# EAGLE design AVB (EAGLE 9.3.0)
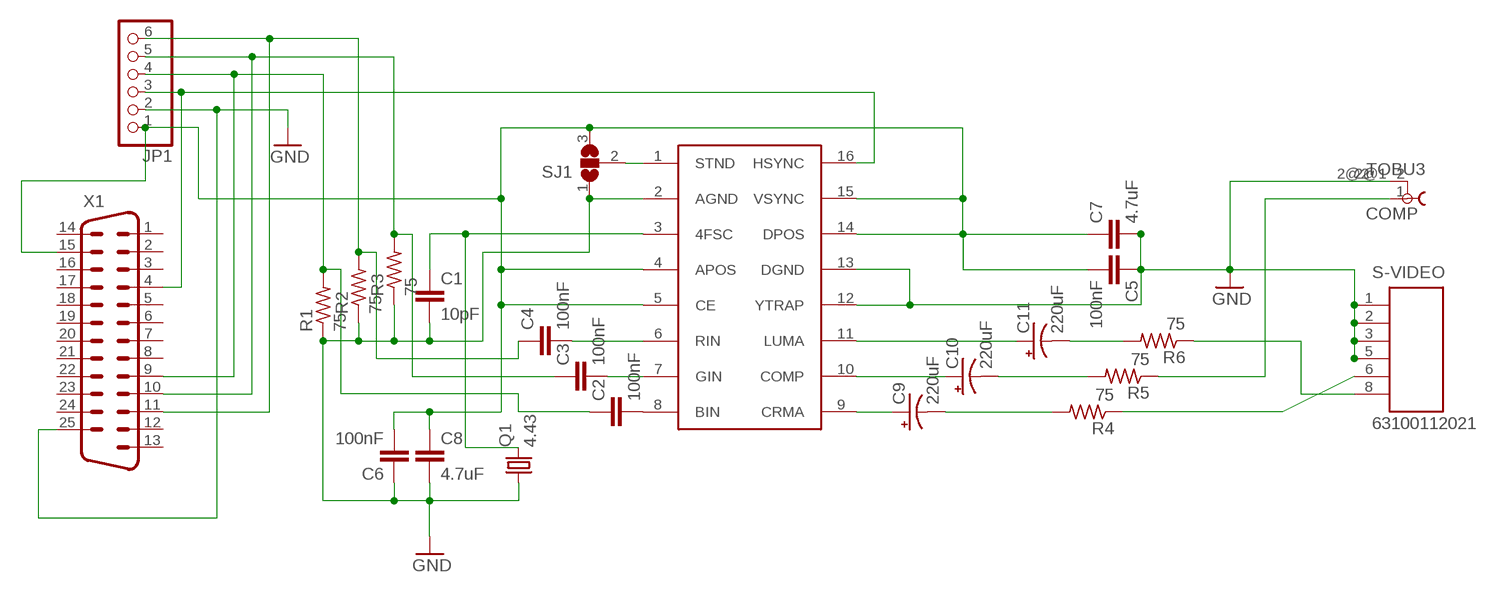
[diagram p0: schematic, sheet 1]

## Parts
C1  10pF  C-EUC0603  [C0603]
C2  100nF  C-EUC0603  [C0603]
C3  100nF  C-EUC0603  [C0603]
C4  100nF  C-EUC0603  [C0603]
C5  100nF  C-EUC0603  [C0603]
C6  100nF  C-EUC0603  [C0603]
C7  4.7uF  C-EUC0603  [C0603]
C8  4.7uF  C-EUC0603  [C0603]
C9  220uF  CPOL-USCT6032  [CT6032]
C10  220uF  CPOL-USCT6032  [CT6032]
C11  220uF  CPOL-USCT6032  [CT6032]
COMP  TOBU3  [TOBU3]
JP1  PINHD-1X6  [1X06]
Q1  4.43  CRYSTALHC49S  [HC49/S]
R1  75  R-US_R0805  [R0805]
R2  75  R-US_R0805  [R0805]
R3  75  R-US_R0805  [R0805]
R4  75  R-US_R0805  [R0805]
R5  75  R-US_R0805  [R0805]
R6  75  R-US_R0805  [R0805]
S-VIDEO  63100112021  [63100112021]
SJ1  SJ2W  [SJ_2]
U1  AD725  [SO16W]
X1  M25D  [M25D]

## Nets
GND: C1.2 C5.1 C6.1 C7.2 C8.2 COMP.2 JP1.2 Q1.1 R1.1 R2.1 R3.1 S-VIDEO.1 S-VIDEO.2 S-VIDEO.3 S-VIDEO.5 SJ1.1 U1.2(AGND) U1.12(YTRAP) U1.13(DGND) X1.25
N$1: C4.1 JP1.6 R2.2 X1.11
N$2: SJ1.2 U1.1(STND)
N$3: C5.2 C6.2 C7.1 C8.1 JP1.1 SJ1.3 U1.4(APOS) U1.5(CE) U1.14(DPOS) U1.15(VSYNC) X1.15
N$4: C4.2 U1.6(RIN)
N$6: JP1.3 U1.16(HSYNC) X1.4
N$7: C3.2 U1.7(GIN)
N$8: C2.2 U1.8(BIN)
N$9: COMP.1 R5.1
N$10: C3.1 JP1.5 R3.2 X1.10
N$11: R6.1 S-VIDEO.8
N$12: R4.1 S-VIDEO.6
N$14: C2.1 JP1.4 R1.2 X1.9
N$18: C1.1 Q1.2 U1.3(4FSC)
N$23: C11.+ U1.11(LUMA)
N$24: C10.+ U1.10(COMP)
N$25: C9.+ U1.9(CRMA)
N$26: C11.- R6.2
N$27: C10.- R5.2
N$28: C9.- R4.2
Unconnected: COMP.2@1 COMP.2@2 X1.1 X1.2 X1.3 X1.5 X1.6 X1.7 X1.8 X1.12 X1.13 X1.14 X1.16 X1.17 X1.18 X1.19 X1.20 X1.21 X1.22 X1.23 X1.24

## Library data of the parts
C1-C8 = resistor:C-EU: CAPACITOR, European symbol
C9-C11 = adafruit:CPOL-US: POLARIZED CAPACITOR, American symbol
COMP = con-hirschmann:TOBU3: Female Cinch CONNECTOR ( RCA Jack )
JP1 = pinhead:PINHD-1X6: PIN HEADER
Q1 = crystal:CRYSTAL: CRYSTAL; OC_FARNELL: 1667008; OC_NEWARK: unknown
R1-R6 = resistor:R-US_: RESISTOR, American symbol
S-VIDEO = Wuerth_Elektronik_eiCan_Communication_Connectors_v2.2:63100112021: WR-COM Horizontal Shielded Mini DIN, 6 Pins
SJ1 = jumper:SJ2W: SMD solder JUMPER
U1 = ad725:AD725
X1 = con-subd:M25: SUB-D; OC_FARNELL: unknown; OC_NEWARK: unknown

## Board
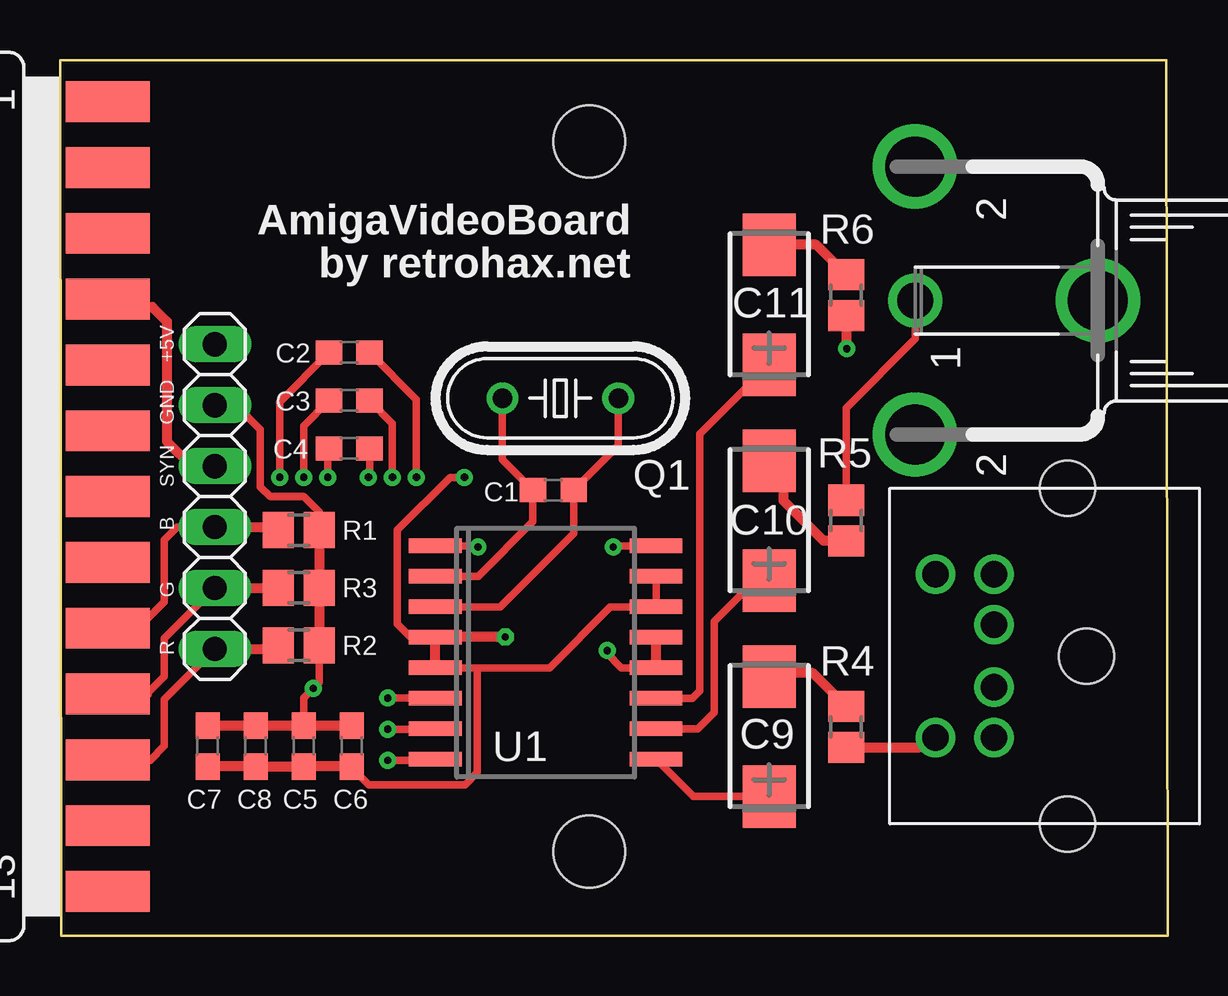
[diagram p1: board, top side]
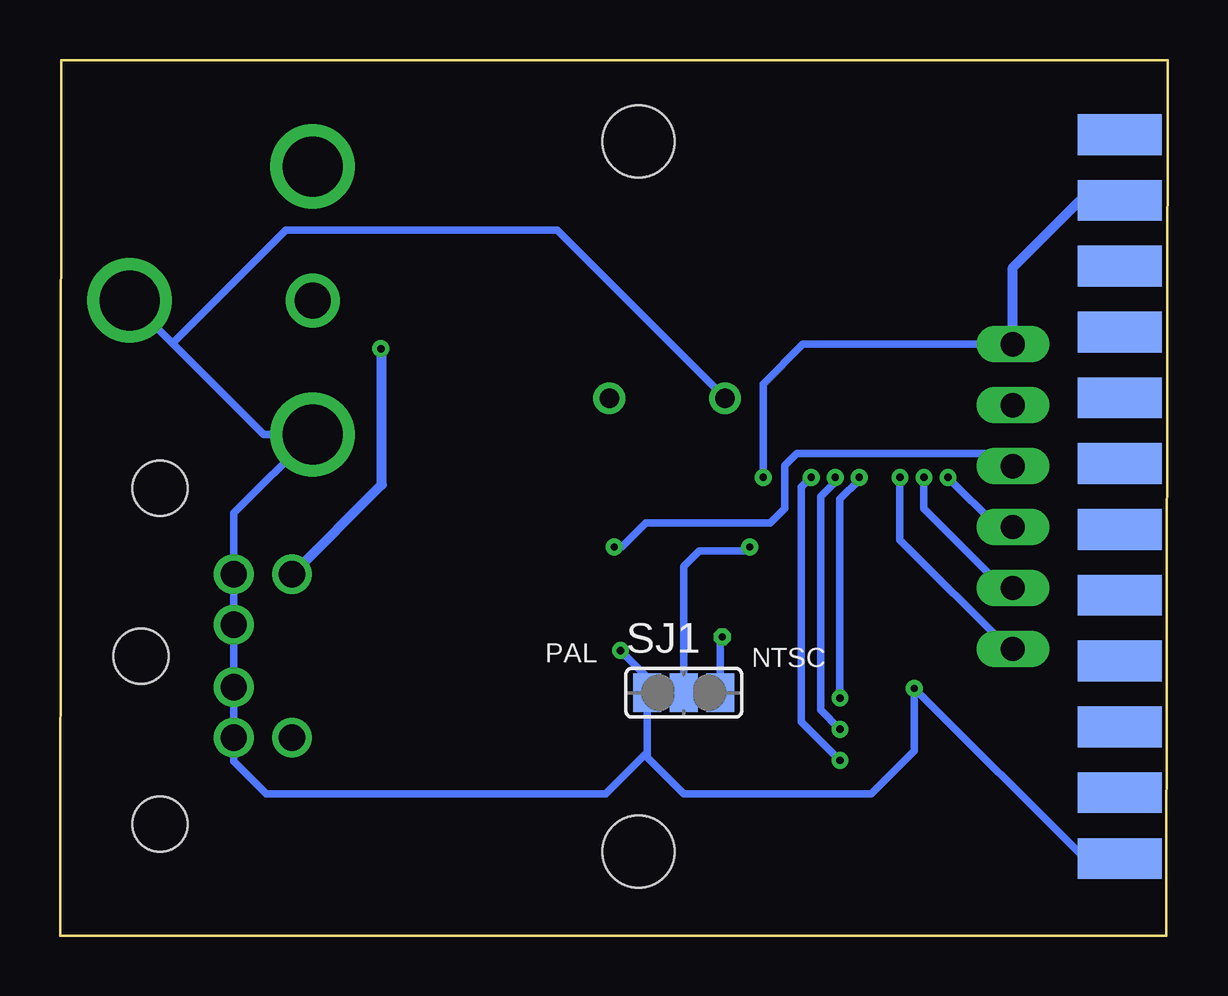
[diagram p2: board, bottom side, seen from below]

Size 46.15 x 36.5 mm. Coordinates in mm from the lower left corner, seen from the top.
Outline: 0.05,0 0,36.5 46.1,36.5 46.15,0 0.05,0
Copper layers (1*16): Top 0.035mm / dielectric 1.5mm / Bottom 0.035mm
Design rules "default": minimum track width 10mil, minimum drill 24mil, track to track 8mil, track to pad 8mil, pad to pad 8mil, via to via 8mil, smd to smd 8mil, copper to edge 40mil, drill to drill 8mil, minimum pad ring 10mil, minimum via ring 8mil, stop-mask expansion 4mil, vias tented up to drill 0mil, thermal gap 10mil
Holes 3 mm at 22.05,33.1 22.05,3.5
Milling: 4 lines

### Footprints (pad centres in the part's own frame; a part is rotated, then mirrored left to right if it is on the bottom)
C0603 = smd 1.1 x 1: 1 -0.85,0; 2 0.85,0
CT6032 = smd 2.6 x 2.2: + 2.5,0; - -2.5,0
TOBU3 = drill 1.5: 1 0,-2.54 | drill 2.5: 2 5.588,-2.54; 2@1 -5.588,-2.54; 2@2 0,5.08
1X06 = drill 1.016 long: 1 -6.35,0; 2 -3.81,0; 3 -1.27,0; 4 1.27,0; 5 3.81,0; 6 6.35,0
HC49/S = drill 0.813: 1 -2.413,0; 2 2.413,0
R0805 = smd 1.3 x 1.5: 1 -0.85,0; 2 0.85,0
63100112021 = drill 1.1: 1 1.3,-8.56; 2 -1.3,-8.56; 3 3.405,-8.56; 5 -3.405,-8.56; 6 3.405,-10.99; 8 -3.405,-10.99 | hole 2.3: -7,-5.49; 0,-4.69; 7,-5.49
SJ_2 = smd 1.168 x 1.6: 1 -1.524,0; 2 0,0; 3 1.524,0
SO16W = smd 0.6 x 2.2: 1 -4.445,-4.6; 2 -3.175,-4.6; 3 -1.905,-4.6; 4 -0.635,-4.6; 5 0.635,-4.6; 6 1.905,-4.6; 7 3.175,-4.6; 8 4.445,-4.6; 9 4.445,4.6; 10 3.175,4.6; 11 1.905,4.6; 12 0.635,4.6; 13 -0.635,4.6; 14 -1.905,4.6; 15 -3.175,4.6; 16 -4.445,4.6
M25D = smd 1.7 x 3.5: 1 16.459,-6.045; 2 13.716,-6.045; 3 10.973,-6.045; 4 8.23,-6.045; 5 5.486,-6.045; 6 2.743,-6.045; 7 0,-6.045; 8 -2.743,-6.045; 9 -5.486,-6.045; 10 -8.23,-6.045; 11 -10.973,-6.045; 12 -13.716,-6.045; 13 -16.459,-6.045 | smd 1.7 x 3.5 bottom: 14 15.088,-6.045; 15 12.344,-6.045; 16 9.601,-6.045; 17 6.858,-6.045; 18 4.115,-6.045; 19 1.372,-6.045; 20 -1.372,-6.045; 21 -4.115,-6.045; 22 -6.858,-6.045; 23 -9.601,-6.045; 24 -12.344,-6.045; 25 -15.088,-6.045

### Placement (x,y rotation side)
C1  20.56,18.57 180 top
C2  12.05,24.3 0 top
C3  12.05,22.3 0 top
C4  12.05,20.3 0 top
C5  10.15,7.9 270 top
C6  12.15,7.9 270 top
C7  6.15,7.9 90 top
C8  8.15,7.9 90 top
C9  29.55,8.3 270 top
C10  29.55,17.3 270 top
C11  29.55,26.3 270 top
COMP  38.17,26.47 270 top
JP1  6.45,18.3 270 top
Q1  20.85,22.4 0 top
R1  9.95,16.9 180 top
R2  9.95,12.1 180 top
R3  9.95,14.5 180 top
R4  32.75,8.7 90 top
R5  32.75,17.3 270 top
R6  32.75,26.7 90 top
S-VIDEO  47.47,11.65 270 top
SJ1  20.16,10.12 0 bottom
U1  20.24,11.8 270 top
X1  -4.05,18.3 90 top

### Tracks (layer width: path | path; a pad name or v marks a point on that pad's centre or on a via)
GND  (via drill 0.3)
  Top 0.305: R2.1 10.8,10.55 v10.55,10.3 10.15,9.9 C5.1 | U1.12 23.39,11.16 22.8,11.75 v22.8,11.88 | R1.1 10.8,17.65 10.15,18.3 8.75,18.3 8.35,18.7 8.35,21.1 7.34,22.11 JP1.2 | U1.2 17.42,14.97 19.71,17.25 C1.2 18.44,19.84 Q1.1
  Top 0.406: 15.62,14.96 U1.2 | 10.51,12.39 R2.1 R3.1 R1.1 | U1.13 U1.12 24.82,11.18 | C6.1 C5.1 C8.2 C7.2
  Bottom 0.254: S-VIDEO.1 38.91,8 | S-VIDEO.2 S-VIDEO.5 | 21.68,10 SJ1.1 21.68,9.8 21.88,9.6
  Bottom 0.305: SJ1.1 21.68,10.76 v22.8,11.88 | X1.25 3.46,3.21 v10.55,10.3 10.55,7.7 12.35,5.9 20.15,5.9 21.68,7.43 21.68,7.63 | 21.68,10 21.68,7.63 | 21.68,7.63 23.42,5.9 37.55,5.9 38.91,7.26 38.91,8 S-VIDEO.3 S-VIDEO.5 38.91,17.61 COMP.2 37.66,20.89 41.51,24.74 | 43.26,26.48 41.51,24.74 | Q1.1 25.44,29.4 36.75,29.4 41.41,24.74 41.51,24.74
  Bottom 0.406: 21.88,9.6 21.88,9.51
N$1  (via drill 0.3)
  Top 0.305: JP1.6 4.35,9.85 4.35,7.9 3.75,7.3 3.72,7.33 X1.11 | C4.1 11.15,20.25 v11.15,19.1
  Top 0.406: JP1.6 9.1,11.95 R2.2
  Bottom 0.305: v11.15,19.1 11.15,16.5 6.6,11.95 JP1.6
N$2  (via drill 0.3)
  Top 0.305: U1.1 17.04,16.24 v17.42,16.2
  Bottom 0.305: SJ1.2 20.16,15.39 19.52,16.02 17.59,16.02 v17.42,16.2
N$3  (via drill 0.3)
  Top 0.254: C5.2 10.15,7.15 | 10.15,7.15 | 17.39,11.16 17.35,11.16
  Top 0.305: U1.15 U1.14 22.94,13.7 20.4,11.16 17.39,11.16 17.39,6.8 16.88,6.29 12.86,6.29 12.15,7 C6.2 | 17.35,11.16 U1.5 | U1.4 14.62,12.43 14.05,13 14.05,16.9 16.25,19.1 v16.85,19.1
  Top 0.406: U1.5 U1.4 | v18.56,12.45 18.27,12.45 18.25,12.44 U1.4 | C7.1 C8.1 10.03,7.05 10.15,7.15 | C6.2 C5.2 | U1.4 16.54,12.43
  Bottom 0.305: SJ1.3 18.64,12.38 v18.56,12.45 | v16.85,19.1 16.85,23 15.2,24.65 JP1.1
  Bottom 0.406: X1.15 3.66,30.64 6.45,27.85 JP1.1
N$4  (via drill 0.3)
  Top 0.305: C4.2 12.9,19.15 v12.85,19.1 | v13.65,9.9 U1.6
  Bottom 0.305: v12.85,19.1 12.85,19 13.65,18.2 v13.65,9.9
N$6  (via drill 0.3)
  Top 0.305: U1.16 23.09,16.24 v23.05,16.2
  Top 0.406: X1.4 2.32,26.2 3.85,26.2 4.45,25.6 4.45,20.6 5.48,19.57 JP1.3
  Bottom 0.305: JP1.3 6.98,20.1 15.45,20.1 15.95,19.6 15.95,17.8 16.55,17.2 21.75,17.2 22.75,16.2 v23.05,16.2
N$7  (via drill 0.3)
  Top 0.305: C3.2 13.85,21.35 v13.85,19.1 | v13.65,8.6 15.61,8.6 U1.7
  Bottom 0.305: v13.85,19.1 13.85,18.9 14.45,18.3 14.45,9.4 v13.65,8.6
N$8  (via drill 0.3)
  Top 0.305: C2.2 14.85,22.35 v14.85,19.1 | U1.8 15.58,7.3 v13.65,7.3
  Bottom 0.305: v13.65,7.3 15.26,8.91 15.26,18.69 v14.85,19.1
N$9
  Top 0.305: COMP.1 35.63,24.88 32.75,22 R5.1
N$10  (via drill 0.3)
  Top 0.305: JP1.5 4.35,12.39 4.35,10.8 3.62,10.07 | C3.1 10.15,21.25 v10.15,19.1
  Top 0.406: JP1.5 R3.2 | 3.62,10.07 X1.10
  Bottom 0.305: v10.15,19.1 10.15,17.8 6.84,14.49 JP1.5
N$11  (via drill 0.3)
  Top 0.406: R6.1 32.75,24.49 v32.78,24.46
  Bottom 0.305: v32.78,24.46 32.73,24.42 | 32.73,24.42
  Bottom 0.406: S-VIDEO.8 32.73,18.8 32.73,24.42
N$12
  Top 0.406: S-VIDEO.6 36.22,8.25 35.83,7.85 R4.1
N$14  (via drill 0.3)
  Top 0.305: JP1.4 4.88,17.03 4.35,16.5 4.35,13.9 3.26,12.81 X1.9 | C2.1 9.15,22.25 v9.15,19.1
  Top 0.406: JP1.4 9.1,17.03 R1.2 | X1.9 2.18,13
  Bottom 0.305: v9.15,19.1 7.08,17.03 JP1.4
N$18
  Top 0.305: U1.3 18.35,13.7 21.4,16.75 C1.1 23.26,20.43 Q1.2
N$23
  Top 0.305: U1.11 26.34,9.89 26.65,10.2 26.65,20.9 C11.+
N$24
  Top 0.305: U1.10 26.57,8.62 27.25,9.3 27.25,13.1 28.96,14.81 29.54,14.81
  Top 0.406: 29.54,14.81 C10.+
N$25
  Top 0.305: U1.9 26.39,5.8 C9.+
N$26
  Top 0.406: C11.- 31.5,28.8 R6.2
N$27
  Top 0.406: R5.2 31.82,16.45 30.15,18.11 30.15,19.2 C10.-
N$28
  Top 0.406: R4.2 31.36,10.94 29.69,10.94 C9.-

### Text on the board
tPlace: +5V | GND | SYN | B | G | R
tNames: AmigaVideoBoard / by retrohax.net
bNames: NTSC | PAL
